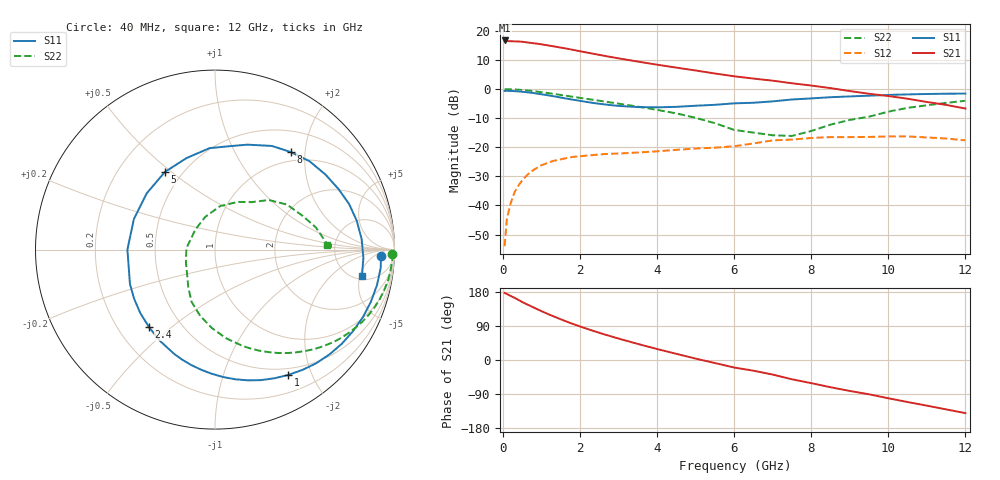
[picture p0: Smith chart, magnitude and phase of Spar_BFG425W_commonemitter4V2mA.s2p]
! Filename: 42bfg425.001
! BFG425W Field C1
! V1=8.013E-001V,V2=4.000E+000V, I1=1.856E-005A, I2=2.000E-003A
# GHz  S  MA  R 50
!  S11  S21  S12  S22
!Freq(GHz)  Mag  Ang  Mag  Ang  Mag  Ang  Mag  Ang
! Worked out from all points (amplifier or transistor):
!   44 points, 40 MHz to 12 GHz, reference 50 ohm
!   highest |S21| = 16.6 dB at 40 MHz (marker M1)
!   |S21| within 3 dB of that: start of sweep to 1.728 GHz
!   unconditionally stable (mu >= 1): 3.114 GHz to end of sweep
!   at 700 MHz: K = 0.19, MSG = 22.2 dB, |S12| = -28.6 dB
!   at 2.4 GHz: K = 0.72, MSG = 17.3 dB, |S12| = -22.6 dB
!   at 12 GHz: K = 1.80, MAG = 0.3 dB, |S12| = -17.7 dB
!   S11 on the Smith chart (normalised r, x): 40 MHz: 21, -10; 1 GHz: 0.41, -1.67; 2.4 GHz: 0.33, -0.42; 5 GHz: 0.40, +0.47; 8 GHz: 0.84, +1.73; 12 GHz: 5.64, -5.40
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0.04  0.925 -2.1  6.795 177.1  0.002 61.4  0.989 -1.4
0.1  0.929 -6.2  6.635 174.2  0.006 80.3  0.989 -3.4
0.2  0.924 -12.3  6.588 168.8  0.011 78.4  0.985 -6.9
0.3  0.916 -18.5  6.557 164.1  0.017 75.7  0.979 -10.2
0.5  0.893 -30.6  6.457 152.9  0.027 68.4  0.958 -16.8
0.8  0.848 -48.3  6.074 138.2  0.041 57.8  0.914 -26.1
1  0.809 -59.7  5.83 128.8  0.049 51.3  0.878 -31.8
1.2  0.771 -70.6  5.54 119.8  0.055 45.4  0.843 -37.2
1.5  0.711 -86.5  5.12 107.3  0.062 37.3  0.788 -44.4
1.8  0.656 -101.8  4.709 95.6  0.068 30.5  0.735 -51.0
2.2  0.594 -121.0  4.185 81.5  0.072 23.2  0.671 -59.1
2.4  0.567 -130.5  3.953 74.9  0.074 20.1  0.641 -62.9
3  0.511 -158.0  3.348 56.5  0.078 12.8  0.559 -73.9
3.5  0.488 180.0  2.945 42.4  0.081 8.4  0.497 -83.0
4.5  0.493 140.4  2.321 16.2  0.09 1.0  0.38 -102.4
5  0.515 122.8  2.073 3.6  0.095 -4.1  0.319 -114.2
6  0.566 93.1  1.649 -19.9  0.104 -14.1  0.198 -142.5
6.5  0.579 83.2  1.505 -28.2  0.116 -11.7  0.178 -155.5
8  0.688 52.2  1.143 -61.1  0.144 -36.1  0.19 106.9
8.5  0.721 43.1  1.033 -71.9  0.149 -45.2  0.244 83.2
10.5  0.806 11.5  0.679 -110.9  0.153 -80.4  0.473 32.1
12  0.832 -10.2  0.461 -140.1  0.131 -112.4  0.627 2.6
